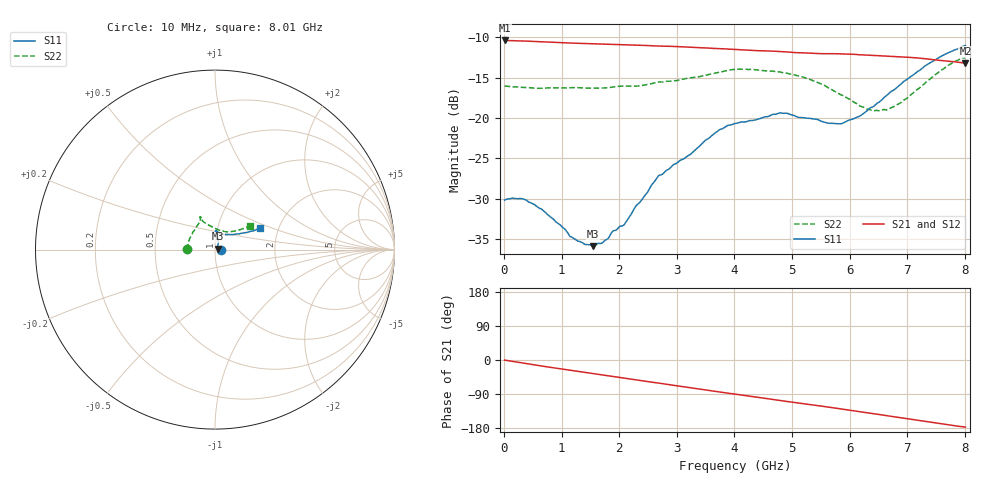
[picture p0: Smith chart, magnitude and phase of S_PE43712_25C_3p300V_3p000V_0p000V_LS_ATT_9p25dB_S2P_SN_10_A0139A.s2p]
! DEVICE ID: PE43712
! File Path: z:\PE43713\PE43713_CHAR_NOM_04292014\AMB\3p300\LS_ATT_9p25dB\PE43713_AMB_3p300V_3p000V_0p000V_LS_ATT_9p25dB_S2P_SN_10_A0139A.s2p
! Serial: 10
! Lot: A0139A
! Temp: 25C
! VDD: 3.300
! VSS: 0.000
! Control_Hi: 3.000
! Control_Lo: 0.000
! Attenuation Step: 9.25dB
! Port 1: RF1
! Port 2: RF2
! ThroughPath:1-2
! IDD: 0.0001469615
! ISS: -7.5e-009
#  Hz  S  RI  R  50
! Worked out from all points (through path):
!   801 points, 10 MHz to 8.01 GHz, reference 50 ohm
!   highest |S21| = -10.41 dB at 10 MHz (marker M1); lowest = -13.2 dB at 8.01 GHz (marker M2)
!   group delay of S21, straight-line fit = 60.8 ps
!   lowest |S11| = -35.9 dB at 1.54 GHz (marker M3), VSWR 1.03, Z = 51.6 + j0.472 ohm
!   |S11| at or under -10 dB: start of sweep to end of sweep
!   |S22| runs from -19.1 to -12.5 dB; largest |S21 - S12| = 0.0011
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1e7  0.031 0.000116  0.3017 -0.00161  0.3018 -0.00165  -0.1578 0.000973
3e8  0.0314 -0.00367  0.297 -0.0393  0.297 -0.0393  -0.154 0.0154
5e8  0.029 -0.00493  0.2908 -0.0636  0.2909 -0.0635  -0.1512 0.0243
9.6e8  0.0217 -0.00339  0.2697 -0.1142  0.2698 -0.1142  -0.1464 0.0461
1.17e9  0.0183 -0.000944  0.2576 -0.1346  0.2576 -0.1347  -0.1434 0.0561
1.35e9  0.0169 0.00112  0.2466 -0.1514  0.2466 -0.1515  -0.1398 0.0634
1.54e9  0.0154 0.00458  0.2336 -0.1681  0.2336 -0.1682  -0.1342 0.073
1.72e9  0.0147 0.00848  0.2205 -0.183  0.2205 -0.183  -0.1297 0.0813
2.09e9  0.0138 0.0171  0.1905 -0.2106  0.1905 -0.2105  -0.1219 0.0994
2.68e9  0.019 0.0394  0.1358 -0.2434  0.1357 -0.2434  -0.0988 0.1344
3.72e9  0.0132 0.0824  0.0292 -0.267  0.029 -0.267  -0.0819 0.1729
4.01e9  0.00986 0.0917  -0.000381 -0.2656  -0.000405 -0.2656  -0.0842 0.1812
4.79e9  0.00483 0.1074  -0.0741 -0.2466  -0.0741 -0.2468  -0.0788 0.1757
5.35e9  0.0154 0.0976  -0.1198 -0.2212  -0.1197 -0.2211  -0.0675 0.1573
5.88e9  0.0385 0.0843  -0.1596 -0.1915  -0.1593 -0.1915  -0.0306 0.1345
6.18e9  0.0606 0.083  -0.1786 -0.1692  -0.1783 -0.1694  -0.0016 0.1185
6.38e9  0.0798 0.0846  -0.1893 -0.1538  -0.189 -0.1538  0.0191 0.1098
6.68e9  0.1129 0.0856  -0.2034 -0.1287  -0.2031 -0.1288  0.0539 0.1001
6.99e9  0.1468 0.0909  -0.215 -0.1012  -0.2147 -0.1012  0.0868 0.0995
7.36e9  0.1908 0.1  -0.2215 -0.0663  -0.2213 -0.0662  0.1307 0.109
7.73e9  0.2293 0.1109  -0.2216 -0.0333  -0.2215 -0.0334  0.1738 0.1241
8.01e9  0.2528 0.1225  -0.2182 -0.0112  -0.2179 -0.0116  0.1952 0.1336
